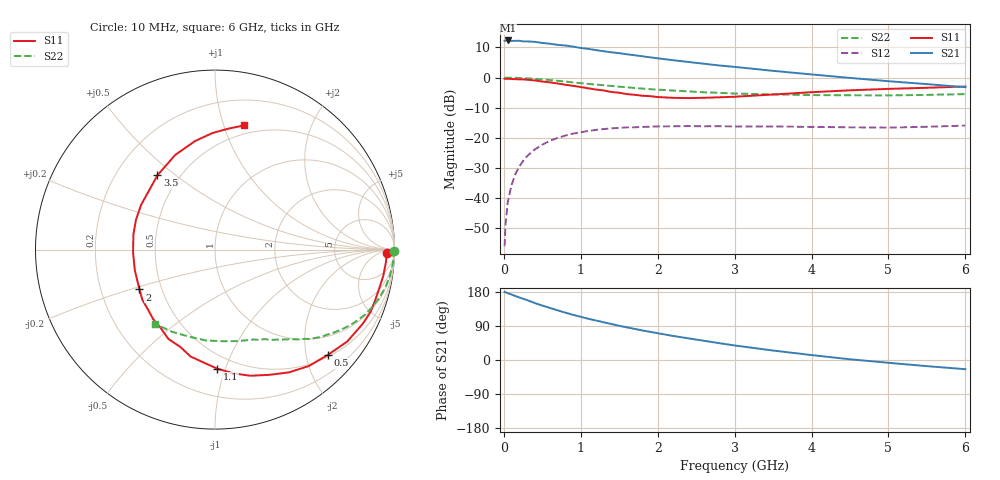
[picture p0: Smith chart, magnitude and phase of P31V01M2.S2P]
! SIEMENS Small Signal Semiconductors
! BFP181
! Si NPN RF Bipolar Junction Transistor in SOT143
! VCE = 1 V  IC = 1.2 mA
! Common Emitter S-Parameters:  March  1996
# GHz  S  MA  R  50
!  f  S11  S21  S12  S22
! GHz  MAG  ANG  MAG  ANG  MAG  ANG  MAG  ANG
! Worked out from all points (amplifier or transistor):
!   36 points, 10 MHz to 6 GHz, reference 50 ohm
!   highest |S21| = 12.3 dB at 50 MHz (marker M1)
!   |S21| within 3 dB of that: start of sweep to 1.148 GHz
!   unconditionally stable (mu >= 1): 2.753 GHz to end of sweep
!   at 250 MHz: K = 0.10, MSG = 19.8 dB, |S12| = -27.7 dB
!   at 1.4 GHz: K = 0.56, MSG = 12.6 dB, |S12| = -16.8 dB
!   at 6 GHz: K = 1.32, MAG = 3.0 dB, |S12| = -15.9 dB
!   S11 on the Smith chart (normalised r, x): 10 MHz: 39, -15; 500 MHz: 0.54, -2.43; 1.1 GHz: 0.40, -0.94; 2 GHz: 0.37, -0.21; 3.5 GHz: 0.38, +0.43; 6 GHz: 0.42, +1.17
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0.01  0.9559 -1.0  4.068 179.6  0.0016 91.0  0.9982 -0.3
0.02  0.9559 -1.8  4.086 179.2  0.0034 89.6  0.9907 -0.8
0.05  0.9549 -4.3  4.128 176.4  0.0085 91.5  0.9949 -2.1
0.1  0.9488 -8.9  4.049 172.7  0.0166 82.4  0.9941 -4.3
0.2  0.9361 -17.6  4.078 165.1  0.0333 78.7  0.9852 -8.5
0.4  0.8972 -34.8  3.92 150.4  0.064 68.1  0.9542 -16.4
0.5  0.8598 -43.1  3.753 143.6  0.077 62.2  0.9322 -20.1
0.6  0.8331 -51.1  3.645 137.3  0.0897 57.5  0.9102 -23.5
0.8  0.7599 -66.7  3.404 124.9  0.1092 49.1  0.8604 -29.5
0.9  0.73 -74.3  3.264 119.2  0.1176 44.7  0.8328 -32.3
1.1  0.6629 -89.0  2.989 108.7  0.1306 37.9  0.7854 -37.1
1.3  0.6109 -102.9  2.733 99.4  0.1401 31.6  0.7454 -41.3
1.5  0.5614 -117.6  2.543 90.3  0.146 26.5  0.7056 -44.8
1.8  0.4999 -138.7  2.255 78.0  0.1519 20.7  0.6576 -49.4
2  0.4756 -152.2  2.087 70.7  0.1551 17.1  0.6323 -52.3
2.2  0.4616 -165.3  1.942 63.5  0.1557 13.8  0.6093 -55.4
2.8  0.4708 159.2  1.589 44.4  0.1563 6.8  0.5592 -64.0
3.5  0.5239 127.7  1.294 25.0  0.1549 1.8  0.5269 -75.2
4  0.5722 112.8  1.128 13.0  0.152 -0.8  0.5127 -84.9
4.5  0.6149 100.4  0.987 1.9  0.1497 -2.4  0.5088 -95.6
5.5  0.6776 83.8  0.779 -16.2  0.1528 -1.0  0.5168 -117.7
6  0.7103 76.9  0.693 -24.3  0.1599 -1.2  0.5319 -129.0
